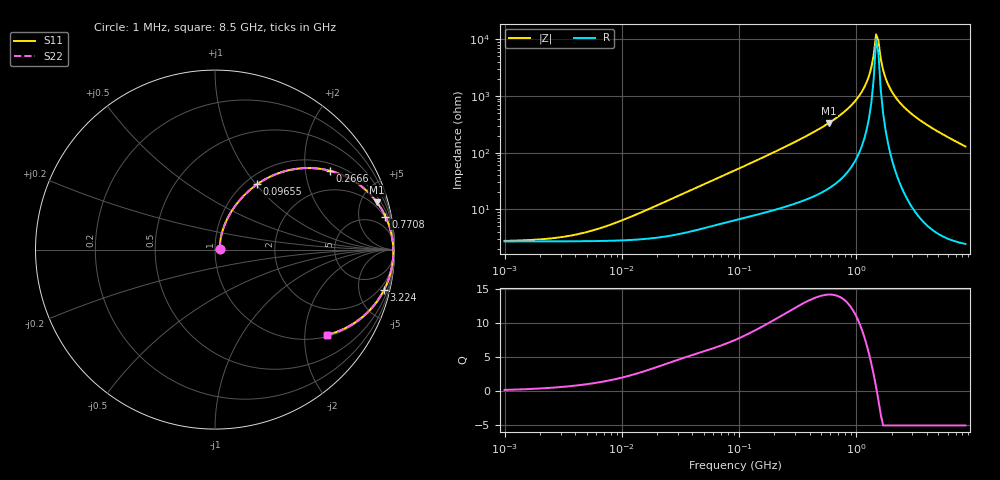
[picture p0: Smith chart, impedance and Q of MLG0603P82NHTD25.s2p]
! S-Parameter Data Generated by TDK Corporation
! Copyright(C) 2025 TDK Corporation.
! All Rights Reserved.
! TDK P/N: MLG0603P82NHTD25 (SMD / SMT Inductor (Coil))
! Property: L=82nH at 300MHz
! Size(LxWxT): 0.6x0.3x0.3mm
! Model Type: s2p (Touchstone File Format Version 1.0)
! Frequency: DC=Yes Start=1MHz Stop=8500MHz 198points Log-sweep
! Model Generated on Feb. 6, 2025
! Terms and conditions regarding TDK Simulation Models:
! 1)This simulation model is being provided solely for informational
!  purposes. Please refer to the specifications of the products in
!  terms of detailed characteristics of such products.
! 2)In no event shall TDK Corporation of any of its subsidiaries be
!  liable for any loss or damage arising, directly or indirectly,
!  from any information contained in this simulation model, including,
!  but not limited to loss or damages arising from any inaccuracies,
!  omissions or errors in connection with such information.
! 3)Any and all copyrights on this simulation model are owned by
!  TDK Corporation.  Duplication or redistribution of this simulation
!  model without prior written permission from TDK Corporation
!  is prohibited.
! 4)This simulation model is subject to any modification or change
!  without any prior notice.
! 5)Neither TDK Corporation nor any of its subsidiaries shall make any
!  warranty, express or implied, including but not limited to the
!  correctness, implied warranties of merchantability and fitness for
!  a particular purpose with respect to this simulation models.
! 6)The use of this simulation model shall be deemed to have consented
!  to the terms and conditions hereof.
! Port Assignments:
!  1 ---@@@--- 2
! Applicable Conditions:
!  Temperature = 25 degC
!  DC Bias Current = 0 A
!  Small Signal Operation
# Hz S MA R 50
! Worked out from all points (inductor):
!   197 points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, 1 MHz to 8.5 GHz, reference 50 ohm
!   read as one part in series: L = 90.1 nH near 15.95 MHz
!   highest Q = 14.2 at 584.3 MHz (marker M1), where L = 91 nH
!   self-resonance near 1.471 GHz
!   S11 on the Smith chart (normalised r, x): 1 MHz: 1.05, +0.01; 96.55 MHz: 1.13, +1.01; 266.6 MHz: 1.23, +2.73; 770.8 MHz: 2, +10; 3.224 GHz: 1.17, -8.40; 8.5 GHz: 1.05, -2.58
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1000000  0.02698 11.6  0.9736 -0.3  0.9736 -0.3  0.02698 11.6
4587603  0.03691 42.4  0.973 -1.5  0.973 -1.5  0.03691 42.4
2.10461e7  0.1187 68.3  0.9625 -6.6  0.9625 -6.6  0.1187 68.3
9.219544e7  0.4177 58.0  0.8553 -24.5  0.8553 -24.5  0.4177 58.0
9.655117e7  0.4323 57.2  0.8477 -25.4  0.8477 -25.4  0.4323 57.2
2.665721e8  0.7774 34.4  0.5665 -50.8  0.5665 -50.8  0.7774 34.4
4.229561e8  0.8902 23.2  0.395 -62.6  0.395 -62.6  0.8902 23.2
5.842944e8  0.9403 16.3  0.2807 -69.7  0.2807 -69.7  0.9403 16.3
7.707615e8  0.9676 11.0  0.1911 -74.8  0.1911 -74.8  0.9676 11.0
1.016736e9  0.984 6.2  0.1086 -78.5  0.1086 -78.5  0.984 6.2
1.222927e9  0.9902 3.2  0.05645 -78.5  0.05645 -78.5  0.9902 3.2
1.34121e9  0.9921 1.7  0.03105 -74.4  0.03105 -74.4  0.9921 1.7
1.404574e9  0.9928 1.0  0.01873 -66.8  0.01873 -66.8  0.9928 1.0
1.470933e9  0.9932 0.3  0.008152 -33.5  0.008152 -33.5  0.9932 0.3
1.540426e9  0.9935 -0.5  0.01052 51.5  0.01052 51.5  0.9935 -0.5
1.613203e9  0.9936 -1.2  0.02203 72.4  0.02203 72.4  0.9936 -1.2
1.689417e9  0.9934 -2.0  0.03456 78.1  0.03456 78.1  0.9934 -2.0
1.940355e9  0.9919 -4.2  0.07346 81.6  0.07346 81.6  0.9919 -4.2
2.444114e9  0.9852 -8.1  0.1415 79.9  0.1415 79.9  0.9852 -8.1
3.224109e9  0.9684 -13.3  0.2304 75.5  0.2304 75.5  0.9684 -13.3
5.115526e9  0.9099 -23.6  0.4008 65.5  0.4008 65.5  0.9099 -23.6
8.5e9  0.7828 -37.4  0.6076 51.5  0.6076 51.5  0.7828 -37.4
